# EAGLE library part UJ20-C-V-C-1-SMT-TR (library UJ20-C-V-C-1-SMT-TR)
USB Connectors USB Jack 2.0, Type-C, Vertical, Copper Alloy, Surface Mount, 6.5H, T&R Source: Datasheet
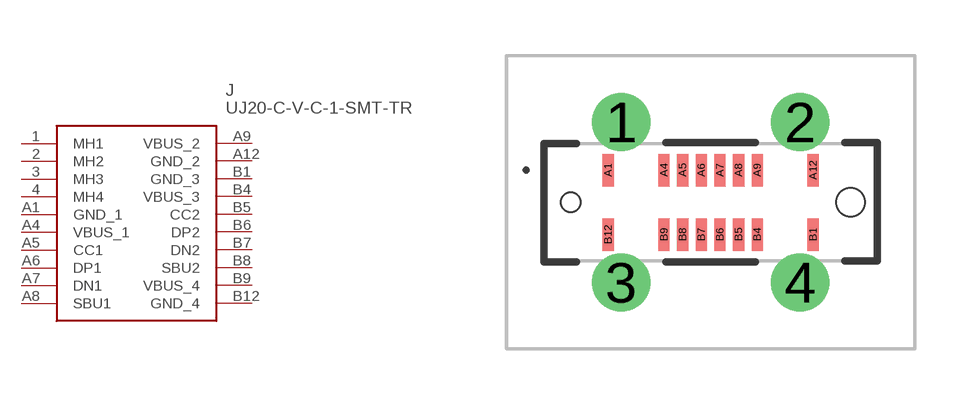
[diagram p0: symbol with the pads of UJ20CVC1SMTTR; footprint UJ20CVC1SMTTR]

Designator prefix J

## UJ20-C-V-C-1-SMT-TR (Description: USB Connectors USB Jack 2.0, Type-C, Vertical, Copper Alloy, Surface Mount, 6.5H, T&R; Height: 6.65mm; Manufacturer_Name: Same Sky; Manufacturer_Part_Number: UJ20-C-V-C-1-SMT-TR; Mouser_Part_Number: 179-UJ20CVC1SMTTR; Mouser_Price-Stock: https://www.mouser.co.uk/ProductDetail/CUI-Devices/UJ20-C-V-C-1-SMT-TR?qs=i8QVZAFTkqRSXXSHLSIhtw%3D%3D)  [UJ20CVC1SMTTR]
1  MH1
2  MH2
3  MH3
4  MH4
A1  GND_1
A4  VBUS_1
A5  CC1
A6  DP1
A7  DN1
A8  SBU1
A9  VBUS_2
A12  GND_2
B1  GND_3
B4  VBUS_3
B5  CC2
B6  DP2
B7  DN2
B8  SBU2
B9  VBUS_4
B12  GND_4

## Footprint UJ20CVC1SMTTR (pad centres in mm)
UJ20-C-V-C-1-SMT-TR-1
drill 1.04 pad 1.56: 1 -2.4,2.15; 2 2.4,2.15; 3 -2.4,-2.15; 4 2.4,-2.15
smd 0.3 x 0.87: A1 -2.75,0.865; A4 -1.25,0.865; A5 -0.75,0.865; A6 -0.25,0.865; A7 0.25,0.865; A8 0.75,0.865; A9 1.25,0.865; A12 2.75,0.865; B1 2.75,-0.865; B4 1.25,-0.865; B5 0.75,-0.865; B6 0.25,-0.865; B7 -0.25,-0.865; B8 -0.75,-0.865; B9 -1.25,-0.865; B12 -2.75,-0.865
hole 0.52 at -3.75,0
hole 0.77 at 3.75,0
